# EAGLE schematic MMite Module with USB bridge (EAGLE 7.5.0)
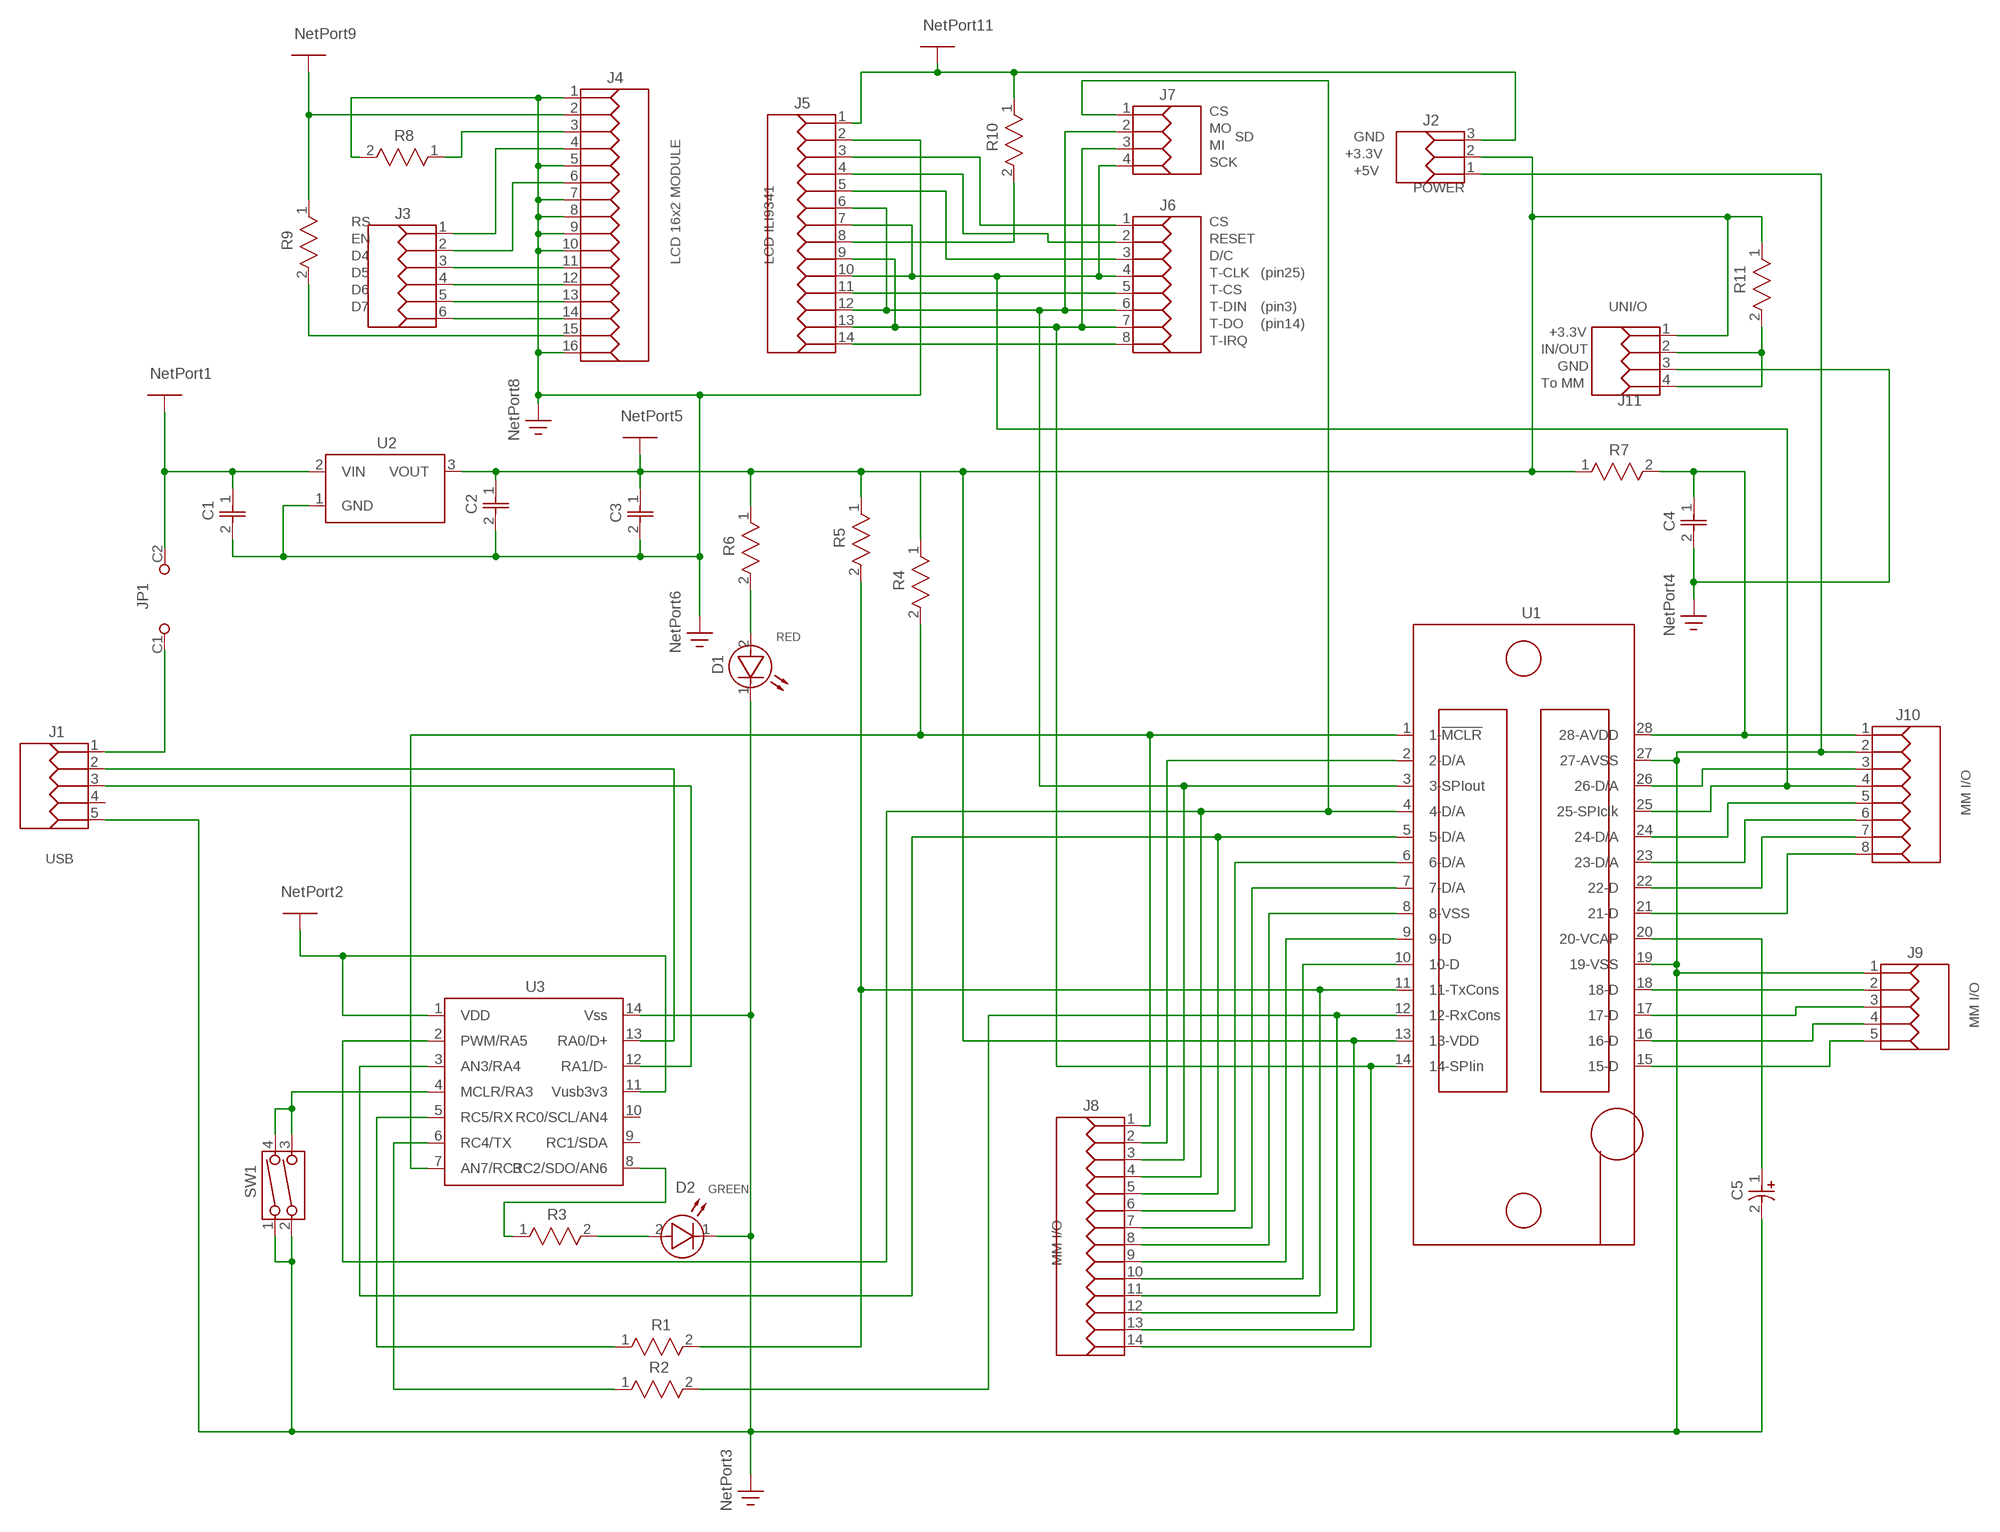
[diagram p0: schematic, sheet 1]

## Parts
C1  10uF  CAP_NONPOLARIZED  [CAP-2.54/4x2.5]
C2  10uF  CAP_NONPOLARIZED  [CAP-2.54/4x2.5]
C3  100nF  CAP_NONPOLARIZED  [CAP-2.54/4x2.5]
C4  100nF  CAP_NONPOLARIZED  [CAP-2.54/4x2.5]
C5  47uF-16V Tan  CAP_POLARIZED1  [CAP-2.54/5.1x2.5]
D1  RED  DIO_LED_2  [LED-5Cil_Red]
D2  GREEN  DIO_LED_2  [LED-5Cil_Red]
J1  MINI_USB  [Mini_USB_51387-578]
J2  HEADER 3F  POWER_I/O  [CON3F]
J3  HEADER 6F  LCD_16X2  [CON6F]
J4  HEADER 16F  LCD_16X2_8  [CON16F]
J5  HEADER 14F  LCD_ILI9341  [CON14F]
J6  HEADER 8F  LCD_ILI9341_5  [CON8F]
J7  HEADER 4F  ILI9341-SD  [CON4F]
J8  HEADER 14F  MM_I/O  [CON14F]
J9  HEADER 5F  MM_I/O_18  [51022-0500]
J10  HEADER 8F  MM_I/O_19  [CON8F]
J11  HEADER 4F  UNI/O-TEMP  [CON4F]
JP1  JUMPER  [JMP]
R1  1K5  RES_FIXED  [RES-10.16/5.1x2.5]
R2  1K5  RES_FIXED  [RES-10.16/5.1x2.5]
R3  1K  RES_FIXED  [RES-10.16/5.1x2.5]
R4  10K  RES_FIXED  [RES-10.16/5.1x2.5]
R5  10K  RES_FIXED  [RES-10.16/5.1x2.5]
R6  1K5  RES_FIXED  [RES-10.16/5.1x2.5]
R7  10R  RES_FIXED  [RES-10.16/5.1x2.5]
R8  1K8  RES_FIXED  [RES-10.16/5.1x2.5]
R9  1K8  RES_FIXED  [RES-10.16/5.1x2.5]
R10  18R  RES_FIXED  [RES-10.16/5.1x2.5]
R11  100K  RES_FIXED  [RES-10.16/5.1x2.5]
SW1  SWITCH  SWITCH_2DIP  [B3F-1]
U1  28pins ZIF  28PINS_ZIF_SOCKET  [28pins_ZIF_pattern]
U2  MCP1700-33  VOLTAGE_REGULATOR  [TO-92]
U3  PIC16F1455  [DIP-14]

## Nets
Net_0: J8.1 R4.2 U1.1(1-!MCLR!) U3.7(AN7/RC3)
Net_1: C1.2 C2.2 C3.2 C4.2 C5.2(MINUS) D1.1(K) D2.1(K) J1.5 J2.1 J4.1 J4.5 J4.7 J4.8 J4.9 J4.10 J4.16 J5.2 J9.1 J10.2 J11.3 R8.2 SW1.1 SW1.2 U1.19(19-VSS) U1.27(27-AVSS) U2.1(GND) U3.14(Vss) ; supply symbol labelled GND
Net_2: C2.1 C3.1 J2.2 J8.13 J11.1 R4.1 R5.1 R6.1 R7.1 R11.1 U1.13(13-VDD) U2.3(VOUT) U3.1(VDD) U3.11(Vusb3v3) ; supply symbol labelled +3V3
Net_3: J7.1 J8.4 U1.4(4-D/A) U3.2(PWM/RA5)
Net_4: J8.5 U1.5(5-D/A) U3.3(AN3/RA4)
Net_5: SW1.3 SW1.4 U3.4(MCLR/RA3)
Net_6: R1.1 U3.5(RC5/RX)
Net_7: J8.11 R1.2 R5.2 U1.11(11-TxCons)
Net_8: R2.1 U3.6(RC4/TX)
Net_9: J8.12 R2.2 U1.12(12-RxCons)
Net_10: R3.1 U3.8(RC2/SDO/AN6)
Net_11: J1.3 U3.12(RA1/D-)
Net_12: D2.2(A) R3.2
Net_13: J1.2 U3.13(RA0/D+)
Net_14: C1.1 J2.3 J4.2 J5.1 JP1.C2 R9.1 R10.1 U2.2(VIN) ; supply symbol labelled +5V
Net_15: C5.1(PLUS) U1.20(20-VCAP)
Net_16: D1.2(A) R6.2
Net_17: C4.1 J10.1 R7.2 U1.28(28-AVDD)
Net_18: J3.1 J4.4
Net_19: J4.3 R8.1
Net_20: J11.2 J11.4 R11.2
Net_21: J3.6 J4.14
Net_22: J3.5 J4.13
Net_23: J3.4 J4.12
Net_24: J3.3 J4.11
Net_25: J3.2 J4.6
Net_26: J4.15 R9.2
Net_27: J9.2 U1.18(18-D)
Net_28: J9.3 U1.17(17-D)
Net_29: J9.4 U1.16(16-D)
Net_30: J9.5 U1.15(15-D)
Net_31: J10.3 U1.26(26-D/A)
Net_32: J5.7 J5.10 J6.4 J7.4 J10.4 U1.25(25-SPIclk)
Net_33: J10.5 U1.24(24-D/A)
Net_34: J10.6 U1.23(23-D/A)
Net_35: J10.7 U1.22(22-D)
Net_36: J10.8 U1.21(21-D)
Net_37: J8.2 U1.2(2-D/A)
Net_38: J5.6 J5.12 J6.6 J7.2 J8.3 U1.3(3-SPIout)
Net_39: J8.6 U1.6(6-D/A)
Net_40: J8.7 U1.7(7-D/A)
Net_41: J8.8 U1.8(8-VSS)
Net_42: J8.9 U1.9(9-D)
Net_43: J8.10 U1.10(10-D)
Net_44: J5.9 J5.13 J6.7 J7.3 J8.14 U1.14(14-SPIin)
Net_45: J5.8 R10.2
Net_46: J1.1 JP1.C1
Net_49: J5.14 J6.8
Net_50: J5.11 J6.5
Net_51: J5.5 J6.3
Net_52: J5.4 J6.2
Net_53: J5.3 J6.1
Unconnected: J1.4 U3.9(RC1/SDA) U3.10(RC0/SCL/AN4)

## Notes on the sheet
- CS
- MO
- SD | GND
- MI
- +3.3V
- SCK
- +5V
- POWER
- RS | CS
- EN | RESET
- D4 | D/C
- D5 | LCD 16x2 MODULE | LCD ILI9341 | T-CLK | (pin25)
- D6 | T-CS
- D7 | T-DIN | (pin3) | UNI/O
- T-DO | (pin14)
- +3.3V
- T-IRQ
- IN/OUT
- GND
- To MM
- RED
- MM I/O
- USB
- MM I/O
- GREEN
- MM I/O

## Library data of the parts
C1 C2 = common:CAP_NONPOLARIZED; DESCRIPTION: Non-polarized
C3 C4 = common:CAP_NONPOLARIZED; DESCRIPTION: Non-polarized; VALUE: 10uF
C5 = common:CAP_POLARIZED1; ATTR_1: Electrolytic; DESCRIPTION: Polarized
D1 = common:DIO_LED_2; DESCRIPTION: LED
D2 = common:DIO_LED_2; DESCRIPTION: LED; VALUE: RED
J1 = common:MINI_USB; DATASHEET: http://datasheets.diptrace.com/con_board_in/510221400_sd.pdf; MANUFACTURER: Molex
J2 = common:POWER_I/O; DATASHEET: http://datasheets.diptrace.com/con_board_in/510221400_sd.pdf; MANUFACTURER: Molex
J3 = common:LCD_16X2
J4 = common:LCD_16X2_8; DATASHEET: http://datasheets.diptrace.com/con_board_in/DF4.pdf; MANUFACTURER: Hirose
J5 = common:LCD_ILI9341
J6 = common:LCD_ILI9341_5; DATASHEET: http://datasheets.diptrace.com/con_board_in/510150300_sd.pdf; MANUFACTURER: Molex
J7 = common:ILI9341-SD; DATASHEET: http://datasheets.diptrace.com/con_board_in/510221400_sd.pdf; MANUFACTURER: Molex
J8 = common:MM_I/O
J9 = common:MM_I/O_18; DATASHEET: http://datasheets.diptrace.com/con_board_in/510221400_sd.pdf; MANUFACTURER: Molex
J10 = common:MM_I/O_19
J11 = common:UNI/O-TEMP; DATASHEET: http://datasheets.diptrace.com/con_board_in/510221400_sd.pdf; MANUFACTURER: Molex
JP1 = common:JUMPER
R1 R2 R6 = common:RES_FIXED; DESCRIPTION: Fixed Resistor
R3-R5 R7-R11 = common:RES_FIXED; DESCRIPTION: Fixed Resistor; VALUE: 1K5
SW1 = common:SWITCH_2DIP; ATTR_1: 2 Positions; DESCRIPTION: DIP Switch
U1 = common:28PINS_ZIF_SOCKET; MANUFACTURER: MICROMITE
U2 = common:VOLTAGE_REGULATOR; DATASHEET: http://datasheets.diptrace.com/microchip/22008d.pdf; MANUFACTURER: Microchip
U3 = common:PIC16F1455; DATASHEET: http://datasheets.diptrace.com/microchip/21203Q.pdf; MANUFACTURER: Microchip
